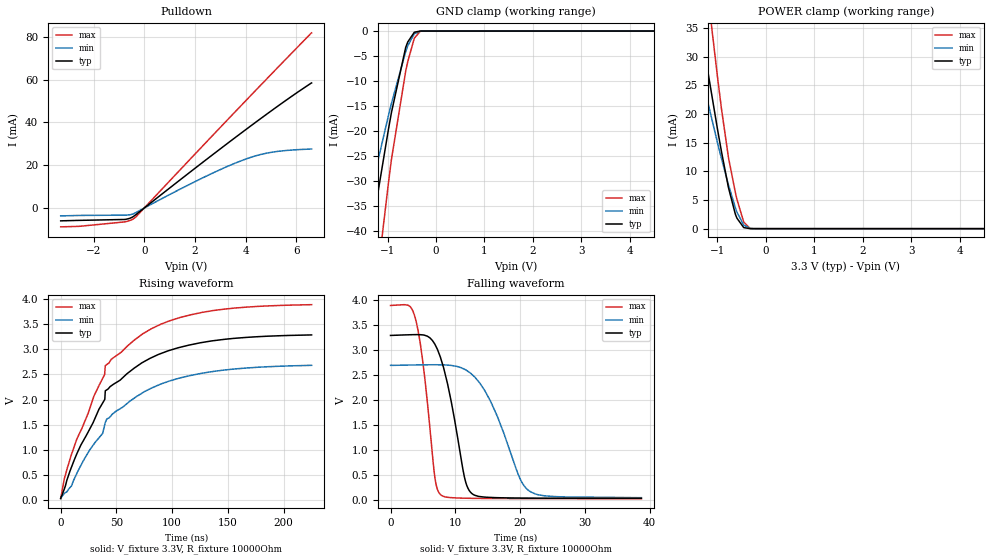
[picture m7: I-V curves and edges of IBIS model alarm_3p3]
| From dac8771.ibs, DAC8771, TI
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|   alarm_3p3 Model
[Model]   alarm_3p3
Model_type   Open_drain
Polarity   Inverting
Vmeas = 1.65
Vref = 3.3
Cref = 2pF
Rref = 10000
|   typ   min   max
|   (nom PVT)   (fast PVT)   (slow PVT)
C_comp   2.401e-12   2.259e-12   2.555e-12
| Where nom  PVT is Nominal Process, 3.3V, 27C
|   Fast PVT is Strong Process,  3.9V, -40C
|   Slow PVT is Weak Process,   2.7V, 150C
[Voltage Range]   3.3   2.7   3.9
|Junction Temperature
[Temperature Range]   27   150   -40
[Pullup Reference]   3.3   2.7   3.9
[Pulldown Reference]   0   0   0
[Power Clamp Reference]   3.3   2.7   3.9
[GND Clamp Reference]   0   0   0
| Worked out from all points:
|   slope of the pulldown table from 0 to 0.495 V, typ, clamps not added: 107 ohm
|   GND clamp passes 1 mA (typ) near -0.50 V on its own axis
|   POWER clamp passes 1 mA (typ) near -0.53 V on its own axis
|   falling waveform, V_fixture 3.3V, R_fixture 10000Ohm: 20-80 % time 2.87ns typ, 4.87ns min, 1.94ns max; typ from 3.3 V to 0.038 V
|   rising waveform, V_fixture 3.3V, R_fixture 10000Ohm: 20-80 % time 56.4ns typ, 59.5ns min, 54.3ns max; typ from 0.035 V to 3.28 V
[Pulldown]
|   Voltage   I(typ)   I(min)   I(max)
-3.3V     -5.996mA   -3.685mA   -8.797mA
-2.577V   -5.776mA   -3.472mA   -8.567mA
-762.3mV  -5.345mA   -3.318mA   -6.468mA
-573.9mV  -4.793mA   -3.162mA   -5.84mA
-390.6mV  -3.615mA   -2.467mA   -4.739mA
2.221V    20.58mA    13.61mA    27.97mA
3.226V    29.68mA    19.16mA    40.49mA
3.99V     36.49mA    22.82mA    49.96mA
4.518V    41.13mA    24.78mA    56.46mA
5.116V    46.3mA     26.21mA    63.81mA
6.6V      58.44mA    27.56mA    81.82mA
[GND Clamp]
|   Voltage   I(typ)   I(min)   I(max)
-3.3V     -543.9mA   -199.1mA   -796.7mA
-2.155V   -90.95mA   -67.61mA   -130.2mA
-1.385V   -43.19mA   -33.67mA   -63.34mA
-983.4mV  -19.7mA    -16.95mA   -30.46mA
-920.7mV  -16.29mA   -14.48mA   -25.69mA
-627mV    -3.29mA    -4.117mA   -8.034mA
-584.1mV  -2.188mA   -2.951mA   -6.107mA
-449.1mV  -241.7uA   -546uA     -1.441mA
-328.2mV  -8.022uA   -38.66uA   -65.61uA
-265.8mV  -981.5nA   -7.935uA   -6.068uA
6.6V      0A         0A         0A
[POWER Clamp]
|   Voltage   I(typ)   I(min)   I(max)
-3.3V     521.4mA    181.5mA    767.4mA
-2.165V   78.74mA    57.99mA    114.2mA
-1.346V   34.88mA    27.24mA    51.55mA
-1.002V   17.48mA    15.08mA    26.66mA
-914.1mV  13.31mA    12.13mA    20.72mA
-772.8mV  7.153mA    7.63mA     12.4mA
-630.3mV  2.519mA    3.649mA    6.31mA
-597.3mV  1.818mA    2.873mA    5.101mA
-456.9mV  181.1uA    614.6uA    1.145mA
-328.2mV  4.701uA    58.57uA    39.34uA
-269.7mV  659nA      16.01uA    4.21uA
6.6V      0A         0A         0A
[Ramp]
R_load = 10000
|   typ   min   max
dV/dt_r   1.95899/5.23766e-08   1.59479/5.58196e-08   2.32158/5.03279e-08
dV/dt_f   1.95905/2.8768e-09   1.5949/4.88531e-09   2.32163/1.93837e-09
[Falling Waveform]
V_fixture = 3.3V
V_fixture_min = 2.7V
V_fixture_max = 3.9V
R_fixture = 10000Ohm
|   Time   V(typ)   V(min)   V(max)
0s        3.3V       2.7V       3.9V
2.979ns   3.314V     2.707V     3.885V
3.959ns   3.316V     2.71V      3.58V
4.99ns    3.31V      2.711V     2.77V
6.797ns   3.135V     2.713V     503.7mV
7.738ns   2.848V     2.711V     109.9mV
11.47ns   429.4mV    2.62V      41.55mV
12.74ns   117.7mV    2.498V     38.8mV
21.26ns   43.3mV     201.6mV    33.92mV
38.72ns   38mV       51.69mV    32.01mV
[Rising Waveform]
V_fixture = 3.3V
V_fixture_min = 2.7V
V_fixture_max = 3.9V
R_fixture = 10000Ohm
|   Time   V(typ)   V(min)   V(max)
0s        34.92mV    41.76mV    30.62mV
3.224ns   221.2mV    137.7mV    425.3mV
9.139ns   625.9mV    271.1mV    875.2mV
22.59ns   1.271V     872.3mV    1.618V
37.61ns   1.93V      1.326V     2.419V
39.58ns   2.004V     1.504V     2.541V
40ns      2.173V     1.543V     2.672V
66.91ns   2.638V     2.041V     3.195V
126.9ns   3.133V     2.522V     3.731V
225.1ns   3.283V     2.679V     3.884V
